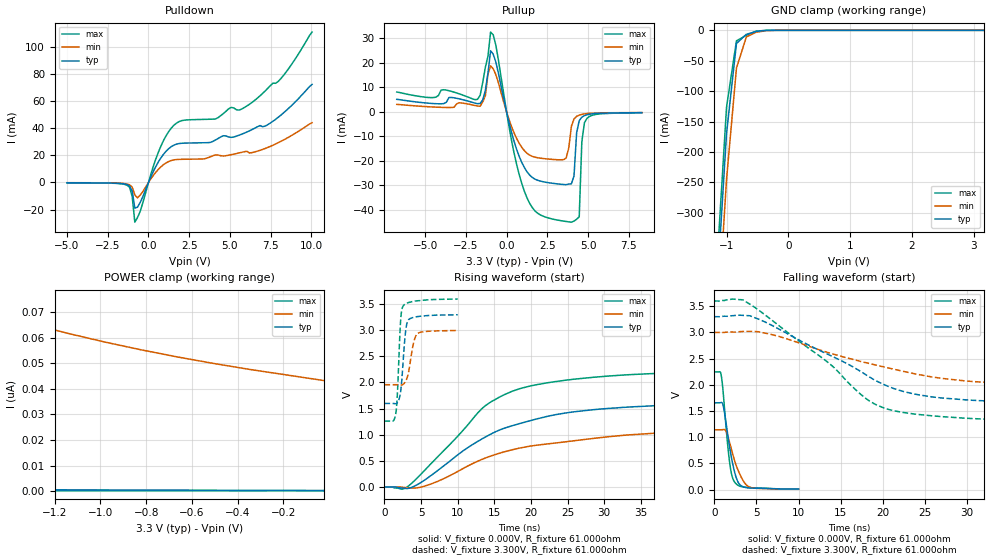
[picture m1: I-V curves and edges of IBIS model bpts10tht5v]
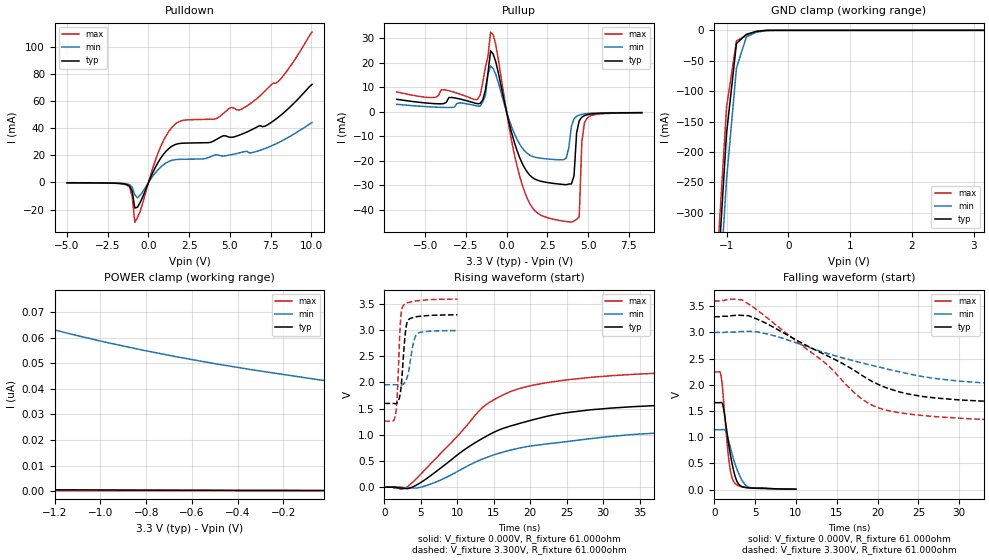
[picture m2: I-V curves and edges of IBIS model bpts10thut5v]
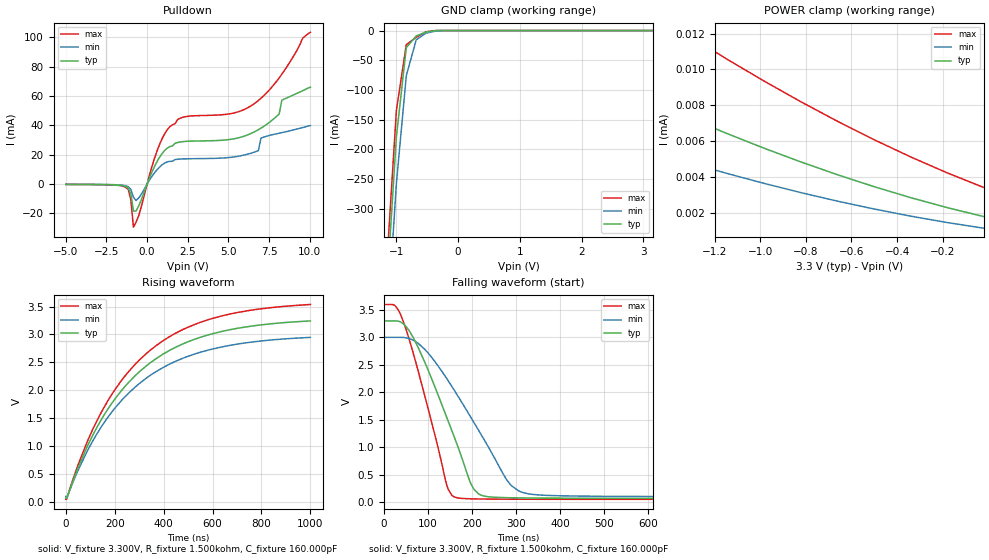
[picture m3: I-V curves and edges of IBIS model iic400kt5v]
[IBIS Ver]  4.0
[File Name]  lpc214x.ibs
[File Rev]  1.0
[Date]   Fri Mar  9 10:51:09 PST 2007
[Source]   Package model from Ansoft Q3D Extractor 7.1.1
[Notes]   IO models Rev 0.20 IBIS Model Design Automation Generation
[Copyright] NXP Semiconductors 2006, 2007. All rights reserved.
|   LPC2141/2142/2144/2146/2148 IBIS Model
[Disclaimer]
| NXP Semiconductors warrants and represents that the IBIS models
| identified herein are owned by NXP Semiconductors (NXP).  The
| models provided are not warranted as fully representing all of the
| operating characteristics and specifications of the semiconductor
| products to which the models relate.  Moreover, unless there is a
| signed, written agreement to the contrary, these models are furnished
| on an "as is" basis without support or warranty of any kind, either
| expressed or implied, regarding the use thereof, and NXP
| specifically disclaims all implied warranties of merchantability and
| fitness of the models for any purpose.
| NXP does not assume any liability arising out of the application
| or use of these IBIS models including infringement of patents and
| copyrights, nor does NXP convey any license under its patents and
| copyrights or the rights of others.
| NXP provides IBIS models as a service to our customers.  You and
| your company shall not distribute, convey, sell, or give these models
| to anyone else without receiving prior written permission from
| NXP.
[Define Package Model]  LQFP64
[Manufacturer]  NXP Semiconductors
[OEM]  NXP Semiconductors
[Description]  LQFP64
|   A full package IBIS Model
|Sim freq : 100 MHz.
|Date : 11/20/06
[Number Of Pins]  64
[Pin Numbers]
pin1   | pin1 = lead1
pin2   | pin2 = lead2
pin3   | pin3 = lead3
pin4   | pin4 = lead4
pin5   | pin5 = lead5
pin6   | pin6 = lead6
pin7   | pin7 = lead7
pin8   | pin8 = lead8
pin9   | pin9 = lead9
pin10   | pin10 = lead10
pin11   | pin11 = lead11
pin12   | pin12 = lead12
pin13   | pin13 = lead13
pin14   | pin14 = lead14
pin15   | pin15 = lead15
pin16   | pin16 = lead16
pin17   | pin17 = lead17
pin18   | pin18 = lead18
pin19   | pin19 = lead19
pin20   | pin20 = lead20
pin21   | pin21 = lead21
pin22   | pin22 = lead22
pin23   | pin23 = lead23
pin24   | pin24 = lead24
pin25   | pin25 = lead25
pin26   | pin26 = lead26
pin27   | pin27 = lead27
pin28   | pin28 = lead28
pin29   | pin29 = lead29
pin30   | pin30 = lead30
pin31   | pin31 = lead31
pin32   | pin32 = lead32
pin33   | pin33 = lead33
pin34   | pin34 = lead34
pin35   | pin35 = lead35
pin36   | pin36 = lead36
pin37   | pin37 = lead37
pin38   | pin38 = lead38
pin39   | pin39 = lead39
pin40   | pin40 = lead40
pin41   | pin41 = lead41
pin42   | pin42 = lead42
pin43   | pin43 = lead43
pin44   | pin44 = lead44
pin45   | pin45 = lead45
pin46   | pin46 = lead46
pin47   | pin47 = lead47
pin48   | pin48 = lead48
pin49   | pin49 = lead49
pin50   | pin50 = lead50
pin51   | pin51 = lead51
pin52   | pin52 = lead52
pin53   | pin53 = lead53
pin54   | pin54 = lead54
pin55   | pin55 = lead55
pin56   | pin56 = lead56
pin57   | pin57 = lead57
pin58   | pin58 = lead58
pin59   | pin59 = lead59
pin60   | pin60 = lead60
pin61   | pin61 = lead61
pin62   | pin62 = lead62
pin63   | pin63 = lead63
pin64   | pin64 = lead64
[Model Data]
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[End Model Data]
[End Package Model]
[Component]   LPC214x
[Manufacturer]  NXP
[Package]
|   typ   min   max
R_pkg   0   0   0  |Values included in pin data
L_pkg   0   0   0  |Values included in pin data
C_pkg   0   0   0  |Values inculded in pin data
[Package Model]  LQFP64
[Pin]   signal_name   model_name   R_pin   L_pin   C_pin
pin1   P0.21   bpts10thut5v   0.1300  4.0559E-9  4.7109E-13
pin2   P0.22   bpts10thut5v   0.1249  3.8553E-9  4.8631E-13
pin3   RTCX1   NC
pin4   P1.19   bpts10thut5v   0.1140  3.4855E-9  4.5269E-13
pin5   RTCX2   NC
pin6   Vss   GND   0.1094  3.2952E-9  4.2167E-13
pin7   V3A   POWER   0.1096  3.2756E-9  4.0402E-13
pin8   P1.18   bpts10thut5v   0.1109  3.2921E-9  3.6808E-13
pin9   P0.25   bpts10thut5v   0.1118  3.3305E-9  3.6694E-013
pin10   D+   usb11f1_iop_hs 0.1126  3.3750E-9  3.9924E-013
pin11   D-   usb11f1_iom_hs 0.1137  3.4080E-9  4.1595E-013
pin12   P1.17   bpts10thut5v   0.1145  3.4513E-9  4.3225E-013
pin13   P0.28   bpts10thut5v   0.1168  3.5314E-9  4.4257E-013
pin14   P0.29   bpts10thut5v   0.1182  3.6136E-9  4.5871E-013
pin15   P0.30   bpts10thut5v   0.1237  3.7941E-9  4.8609E-013
pin16   P1.16   bpts10thut5v   0.1315  4.0543E-9  4.7834E-013
pin17   P0.31OUT   bpts10thut5v   0.1361  4.2525E-9  4.7909E-013
pin18   Vss   GND   0.1370  4.1605E-9  4.9716E-013
pin19   P0.0   bpts10tht5v   0.1359  4.0491E-9  4.5395E-013
pin20   P1.31   bpts10thut5v   0.1359  3.9977E-9  4.7025E-013
pin21   P0.1   bpts10thut5v   0.1368  3.9780E-9  4.6287E-013
pin22   P0.2   iic400kt5v   0.1382  3.9645E-9  4.3275E-013
pin23   V3   POWER   0.1399  3.9938E-9  4.8661E-013
pin24   P1.26   bpts10thut5v   0.1388  3.9783E-9  3.8793E-013
pin25   Vss   GND   0.0849  3.5754E-9  4.5025E-013
pin26   P0.3   iic400kt5v   0.1414  3.9773E-9  4.4598E-013
pin27   P0.4   bpts10thut5v   0.1385  3.9806E-9  4.5362E-013
pin28   P1.25   bpts10thut5v   0.1369  3.9926E-9  4.6653E-013
pin29   P0.5   bpts10thut5v   0.1365  4.0288E-9  4.7531E-013
pin30   P0.6   bpts10thut5v   0.1365  4.0916E-9  4.8687E-013
pin31   P0.7   bpts10thut5v   0.1378  4.1971E-9  4.9554E-013
pin32   P1.24   bpts10thut5v   0.1365  4.2816E-9  4.7853E-013
pin33   P0.8   bpts10thut5v   0.1310  4.0617E-9  4.7309E-013
pin34   P0.9   bpts10thut5v   0.1259  3.8617E-9  4.8581E-013
pin35   P0.10   bpts10thut5v   0.1201  3.6800E-9  4.6639E-013
pin36   P1.23   bpts10thut5v   0.1153  3.5257E-9  4.4746E-013
pin37   P0.11   iic400kt5v   0.1112  3.4101E-9  4.3180E-013
pin38   P0.12   bpts10thut5v   0.1100  3.3561E-9  4.1423E-013
pin39   P0.13   bpts10thut5v   0.1088  3.3002E-9  3.9779E-013
pin40   P1.22   bpts10thut5v   0.1078  3.2747E-9  3.6621E-013
pin41   P0.14   iic400kt5v   0.1076  3.2745E-9  3.6517E-013
pin42   Vss   GND   0.1075  3.2751E-9  3.9548E-013
pin43   V3   POWER   0.1077  3.3057E-9  4.0838E-013
pin44   P1.21   bpts10thut5v   0.1062  3.3049E-9  4.2204E-013
pin45   P0.15   bpts10thut5v   0.1080  3.3717E-9  4.3944E-013
pin46   P0.16   bpts10thut5v   0.1130  3.5156E-9  4.6433E-013
pin47   P0.17   bpts10tht5v   0.1208  3.7554E-9  4.8898E-013
pin48   P1.20   bpts10thut5v   0.1286  4.0340E-9  4.7542E-013
pin49   Vbat   POWER   0.1344  4.2556E-9  4.7786E-013
pin50   Vss   GND   0.1352  4.1540E-9  4.9213E-013
pin51   V3   POWER   0.0836  3.6217E-9  5.4270E-013
pin52   P1.30   bpts10thut5v   0.1370  3.9777E-9  4.7969E-013
pin53   P0.18   bpts10tht5v   0.1349  3.9992E-9  4.5890E-013
pin54   P0.19   bpts10tht5v   0.1360  3.9699E-9  4.5111E-013
pin55   P0.20   bpts10thut5v   0.1381  3.9661E-9  4.4458E-013
pin56   P1.29   bpts10thut5v   0.1408  4.0072E-9  4.2053E-013
pin57   !RESET   bpts10thut5v   0.1433  4.0992E-9  4.1128E-013
pin58   P0.23   bpts10tht5v   0.1380  3.9903E-9  4.3123E-013
pin59   VssA   GND   0.1360  3.9632E-9  4.5084E-013
pin60   P1.28   bpts10thut5v   0.1345  3.9588E-9  4.6165E-013
pin61   XTAL2   NC
pin62   XTAL1   NC
pin63   Vref   POWER   0.1338  4.1409E-9  4.9198E-013
pin64   P1.27   bpts10thut5v   0.1358  4.2774E-9  4.8196E-013
| Models and submodels in the file (5): bpts10tht5v (I/O), bpts10thut5v (I/O), iic400kt5v (I/O_open_drain), usb11f1_iom_hs (I/O), usb11f1_iop_hs (I/O)
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| *   bpts10tht5v  Model   *
[Model]   bpts10tht5v
Model_type   I/O
Polarity   Non-Inverting
Enable   Active-Low
|  Reciever Thresholds
Vinl   = 0.545VV
Vinh   = 1.265VV
| AC Test Load Conditions
Vref   = 0
Cref   = 1.2e-11
Rref   = 1000000000
Vmeas   = 1.4
| [Process Range]   typical   min   max
| C_comp edge width   400.000ps   400.000ps   400.000ps
| C_comp Tstrobe   4.000ps   4.000ps   4.000ps
C_comp   2.882pF   2.754pF   3.016pF
[Temperature Range]   25   125   -40
[Voltage Range]   3.30V   3.00V   3.60V
[GND Clamp Reference]   0.00V   0.00V   0.00V
[Pulldown Reference]   0.00V   0.00V   0.00V
[POWER Clamp Reference]   3.30V   3.00V   3.60V
[Pullup Reference]   3.30V   3.00V   3.60V
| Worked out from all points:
|   slope of the pulldown table from 0 to 0.495 V, typ, clamps not added: 38.6 ohm
|   slope of the pullup table from 0 to 0.495 V, typ, clamps not added: 38.7 ohm
|   GND clamp passes 1 mA (typ) near -0.44 V on its own axis
|   rising waveform, V_fixture 0.000V, R_fixture 61.000ohm: 20-80 % time 13.9ns typ, 18.1ns min, 10.5ns max; typ from 0 V to 1.65 V
|   falling waveform, V_fixture 0.000V, R_fixture 61.000ohm: 20-80 % time 1.06ns typ, 1.41ns min, 788ps max; typ from 1.66 V to 0.008 V
|   rising waveform, V_fixture 3.300V, R_fixture 61.000ohm: 20-80 % time 569ps typ, 787ps min, 437ps max; typ from 1.6 V to 3.29 V
|   falling waveform, V_fixture 3.300V, R_fixture 61.000ohm: 20-80 % time 12.2ns typ, 15ns min, 10.4ns max; typ from 3.3 V to 1.6 V
[GND Clamp]
| ref voltage   0.00V   0.00V   0.00V
|   Voltage   I(typ)   I(min)   I(max)
-5V       -7.936A    -7.958A    -7.931A
-1.16V    -433.2mA   -505.8mA   -392.3mA
-1V       -169.3mA   -244.9mA   -126mA
-840mV    -21.65mA   -62.12mA   -17.29mA
-680mV    -6.579mA   -10.88mA   -8.151mA
-520mV    -1.841mA   -3.127mA   -1.366mA
-360mV    -58.55uA   -596.5uA   -10.53uA
3.16V     300.3pA    45.14nA    134.1pA
[Power Clamp]   | Vtable = Vcc - Vpad
| ref voltage   3.30V   3.00V   3.60V
|   Voltage   I(typ)   I(min)   I(max)
-6.74V    16.52nA    857.8nA    1.18nA
-6.26V    12.33nA    692.5nA    963.8pA
-5.78V    8.96nA     546.5nA    798.2pA
-5.3V     6.516nA    429.9nA    680.5pA
-4.82V    4.749nA    337.5nA    594.2pA
-3.54V    2.1nA      176.9nA    442.2pA
-1.78V    781.7pA    78.68nA    301.1pA
-1.62V    721.7pA    73.79nA    289.6pA
-1.3V     618pA      65.31nA    266.9pA
-820mV    494.3pA    55.22nA    233.5pA
-500mV    427.7pA    49.86nA    211.6pA
-20mV     328.1pA    43.23nA    160.9pA
[Pulldown]
| ref voltage   0.00V   0.00V   0.00V
|   Voltage   I(typ)   I(min)   I(max)
-5V       -226.8uA   -172uA     -259.4uA
-1.32V    -1.578mA   -1.108mA   -2.063mA
-1V       -6.341mA   -3.477mA   -10.45mA
-840mV    -18.89mA   -9.1mA     -29.38mA
-520mV    -15.05mA   -9.482mA   -21.77mA
600mV     15.09mA    9.63mA     22.21mA
1.56V     27.63mA    16.73mA    42.32mA
4.12V     31.49mA    20.45mA    47.01mA
5.08V     33.37mA    20.55mA    55.52mA
6.2V      38.22mA    21.8mA     57.89mA
8.12V     49.75mA    30.36mA    76.76mA
10.04V    72.56mA    44.23mA    111.2mA
[Pullup]   | Vtable = Vcc - Vpad
| ref voltage   3.30V   3.00V   3.60V
|   Voltage   I(typ)   I(min)   I(max)
-6.74V    5.102mA    3.047mA    8.092mA
-1.78V    3.316mA    2.358mA    5.11mA
-1.3V     8.752mA    6.618mA    18.2mA
-980mV    24.92mA    18.76mA    32.55mA
460mV     -12.04mA   -8.591mA   -16.77mA
1.26V     -24.51mA   -16.93mA   -35.2mA
3.5V      -29.67mA   -19.53mA   -44.61mA
3.98V     -29.41mA   -5.895mA   -45.06mA
4.46V     -3.621mA   -1.331mA   -42.82mA
4.62V     -2.179mA   -1.037mA   -12.26mA
4.94V     -1.193mA   -714.9uA   -2.614mA
8.3V      -339.1uA   -299.2uA   -399.9uA
[Ramp]
R_load   = 61.000ohm
|   dV/dt(typ)   dV/dt(min)   dV/dt(max)
dV/dt_r   305.900mV/3.510ns   145.145mV/2.850ns   490.517mV/4.045ns
dV/dt_f   219.141mV/3.115ns   95.446mV/2.510ns   385.597mV/3.650ns
[Rising Waveform]  | cubic spline decimation from 16001 points
V_fixture   = 0.000V
R_fixture   = 61.000ohm
|   Time   V(typ)   V(min)   V(max)
0s        2.719nV    462.7nV    1.218nV
2.365ns   -18.26mV   -1.462mV   -40.39mV
3.085ns   -29.34mV   -13.19mV   2.008mV
6.465ns   232.4mV    64.83mV    463.4mV
13.75ns   954.3mV    553.4mV    1.553V
17.31ns   1.167V     708.3mV    1.824V
20.09ns   1.276V     786.4mV    1.937V
25.98ns   1.44V      886.4mV    2.063V
37.81ns   1.561V     1.037V     2.177V
80ns      1.65V      1.132V     2.242V
[Falling Waveform]  | cubic spline decimation from 2001 points
V_fixture   = 0.000V
R_fixture   = 61.000ohm
|   Time   V(typ)   V(min)   V(max)
0s        1.656V     1.141V     2.245V
815ps     1.661V     1.141V     2.196V
1.14ns    1.544V     1.146V     1.714V
1.44ns    1.234V     1.103V     1.128V
1.775ns   861.6mV    927.3mV    589.7mV
2.07ns    588.3mV    751mV      285.4mV
2.43ns    326.3mV    545.9mV    139.7mV
3.07ns    88.13mV    281.3mV    62.36mV
4.29ns    29.3mV     41.45mV    33.11mV
10ns      7.585mV    7.934mV    6.746mV
[Rising Waveform]  | cubic spline decimation from 2001 points
V_fixture   = 3.300V
V_fixture_min = 3.000V
V_fixture_max = 3.600V
R_fixture   = 61.000ohm
|   Time   V(typ)   V(min)   V(max)
0s        1.598V     1.956V     1.261V
1.545ns   1.593V     1.956V     1.409V
1.73ns    1.608V     1.956V     1.697V
2.195ns   1.813V     1.95V      3.166V
2.505ns   2.318V     1.96V      3.451V
2.91ns    3.005V     2.029V     3.505V
3.29ns    3.199V     2.198V     3.526V
4.025ns   3.244V     2.786V     3.551V
4.51ns    3.258V     2.932V     3.56V
10ns      3.293V     2.992V     3.593V
[Falling Waveform]  | cubic spline decimation from 16001 points
V_fixture   = 3.300V
V_fixture_min = 3.000V
V_fixture_max = 3.600V
R_fixture   = 61.000ohm
|   Time   V(typ)   V(min)   V(max)
0s        3.3V       3V         3.6V
3.445ns   3.325V     3.018V     3.619V
7.415ns   3.086V     2.935V     3.162V
13.46ns   2.584V     2.618V     2.432V
18.01ns   2.189V     2.421V     1.736V
19.39ns   2.06V      2.368V     1.604V
21.92ns   1.896V     2.275V     1.485V
26.97ns   1.748V     2.123V     1.392V
37.59ns   1.661V     2.009V     1.313V
80ns      1.602V     1.959V     1.263V
| bpts10thut5v
|   Bidirectional Pad
|   Plain Input
|   3state Output
|   10 ns Slew Rate Control
|   TTL with Hystersis
|   Pull Up
|   5 V Tolerant
[Model]   bpts10thut5v
Model_type   I/O
Polarity   Non-Inverting
Enable   Active-Low
|  Reciever Thresholds
Vinl   = 0.545VV
Vinh   = 1.265VV
| AC Test Load Conditions
Vref   = 0
Cref   = 1.2e-11
Rref   = 1000000000
Vmeas   = 1.4
| [Process Range]   typical   min   max
| C_comp edge width   400.000ps   400.000ps   400.000ps
| C_comp Tstrobe   4.000ps   4.000ps   4.000ps
C_comp   2.882pF   2.755pF   3.017pF
[Temperature Range]   25   125   -40
[Voltage Range]   3.30V   3.00V   3.60V
[GND Clamp Reference]   0.00V   0.00V   0.00V
[Pulldown Reference]   0.00V   0.00V   0.00V
[POWER Clamp Reference]   3.30V   3.00V   3.60V
[Pullup Reference]   3.30V   3.00V   3.60V
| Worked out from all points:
|   slope of the pulldown table from 0 to 0.495 V, typ, clamps not added: 38.6 ohm
|   slope of the pullup table from 0 to 0.495 V, typ, clamps not added: 38.7 ohm
|   GND clamp passes 1 mA (typ) near -0.44 V on its own axis
|   rising waveform, V_fixture 0.000V, R_fixture 61.000ohm: 20-80 % time 13.9ns typ, 18ns min, 10.4ns max; typ from 0.001 V to 1.65 V
|   falling waveform, V_fixture 0.000V, R_fixture 61.000ohm: 20-80 % time 1.06ns typ, 1.42ns min, 789ps max; typ from 1.66 V to 0.009 V
|   rising waveform, V_fixture 3.300V, R_fixture 61.000ohm: 20-80 % time 568ps typ, 786ps min, 435ps max; typ from 1.6 V to 3.29 V
|   falling waveform, V_fixture 3.300V, R_fixture 61.000ohm: 20-80 % time 12.2ns typ, 15ns min, 10.4ns max; typ from 3.3 V to 1.6 V
[GND Clamp]
| ref voltage   0.00V   0.00V   0.00V
|   Voltage   I(typ)   I(min)   I(max)
-5V       -7.936A    -7.958A    -7.931A
-1.16V    -433.2mA   -505.8mA   -392.3mA
-1V       -169.3mA   -244.9mA   -126mA
-840mV    -21.68mA   -62.13mA   -17.32mA
-680mV    -6.6mA     -10.9mA    -8.182mA
-520mV    -1.87mA    -3.149mA   -1.413mA
-360mV    -102.1uA   -619.8uA   -80.45uA
3.16V     297.4pA    45.14nA    130.5pA
[Power Clamp]   | Vtable = Vcc - Vpad
| ref voltage   3.30V   3.00V   3.60V
|   Voltage   I(typ)   I(min)   I(max)
-6.74V    16.53nA    857.8nA    1.186nA
-6.26V    12.34nA    692.5nA    969.7pA
-5.78V    8.966nA    546.5nA    803.5pA
-5.3V     6.521nA    429.9nA    685.1pA
-4.82V    4.753nA    337.5nA    598.2pA
-3.54V    2.102nA    176.9nA    444.5pA
-1.78V    781.9pA    78.68nA    301.1pA
-1.62V    721.7pA    73.79nA    289.4pA
-1.3V     617.5pA    65.31nA    266.3pA
-820mV    493.2pA    55.22nA    232.2pA
-500mV    426pA      49.86nA    209.8pA
-20mV     325.5pA    43.23nA    158.2pA
[Pulldown]
| ref voltage   0.00V   0.00V   0.00V
|   Voltage   I(typ)   I(min)   I(max)
-5V       -226.8uA   -172uA     -259.4uA
-1.32V    -1.578mA   -1.108mA   -2.063mA
-1V       -6.341mA   -3.477mA   -10.45mA
-840mV    -18.89mA   -9.1mA     -29.38mA
-520mV    -15.05mA   -9.482mA   -21.77mA
600mV     15.09mA    9.63mA     22.21mA
1.56V     27.63mA    16.73mA    42.32mA
4.12V     31.49mA    20.45mA    47.01mA
5.08V     33.37mA    20.55mA    55.52mA
6.2V      38.22mA    21.8mA     57.89mA
8.12V     49.75mA    30.36mA    76.76mA
10.04V    72.56mA    44.23mA    111.2mA
[Pullup]   | Vtable = Vcc - Vpad
| ref voltage   3.30V   3.00V   3.60V
|   Voltage   I(typ)   I(min)   I(max)
-6.74V    5.102mA    3.047mA    8.092mA
-1.78V    3.316mA    2.358mA    5.11mA
-1.3V     8.752mA    6.618mA    18.2mA
-980mV    24.92mA    18.76mA    32.55mA
460mV     -12.04mA   -8.591mA   -16.77mA
1.26V     -24.51mA   -16.93mA   -35.2mA
3.5V      -29.67mA   -19.53mA   -44.61mA
3.98V     -29.41mA   -5.895mA   -45.06mA
4.46V     -3.621mA   -1.331mA   -42.82mA
4.62V     -2.179mA   -1.037mA   -12.26mA
4.94V     -1.193mA   -714.9uA   -2.614mA
8.3V      -339.1uA   -299.2uA   -399.9uA
[Ramp]
R_load   = 61.000ohm
|   dV/dt(typ)   dV/dt(min)   dV/dt(max)
dV/dt_r   306.458mV/3.515ns   145.450mV/2.865ns   491.498mV/4.055ns
dV/dt_f   219.141mV/3.115ns   95.446mV/2.510ns   385.597mV/3.650ns
[Rising Waveform]  | cubic spline decimation from 16001 points
V_fixture   = 0.000V
R_fixture   = 61.000ohm
|   Time   V(typ)   V(min)   V(max)
0s        970.7uV    817.2uV    1.159mV
2.365ns   -17.13mV   -644.9uV   -37.02mV
3.215ns   -25.21mV   -13.15mV   18.29mV
6.515ns   239.9mV    69.07mV    474mV
13.58ns   943.6mV    545.7mV    1.538V
17.24ns   1.167V     707.4mV    1.824V
20.38ns   1.289V     794.1mV    1.949V
28.18ns   1.477V     925.9mV    2.096V
37.37ns   1.56V      1.035V     2.177V
80ns      1.652V     1.133V     2.244V
[Falling Waveform]  | cubic spline decimation from 2001 points
V_fixture   = 0.000V
R_fixture   = 61.000ohm
|   Time   V(typ)   V(min)   V(max)
0s        1.659V     1.142V     2.247V
815ps     1.663V     1.142V     2.198V
1.11ns    1.572V     1.147V     1.776V
1.41ns    1.27V      1.115V     1.188V
1.78ns    859.1mV    926mV      587mV
2.045ns   612mV      767.6mV    306.8mV
2.435ns   325.7mV    545.2mV    142.9mV
2.995ns   103.8mV    311.2mV    71.31mV
4.125ns   34.19mV    54.7mV     39.1mV
10ns      8.903mV    9.047mV    8.293mV
[Rising Waveform]  | cubic spline decimation from 2001 points
V_fixture   = 3.300V
V_fixture_min = 3.000V
V_fixture_max = 3.600V
R_fixture   = 61.000ohm
|   Time   V(typ)   V(min)   V(max)
0s        1.6V       1.956V     1.263V
1.545ns   1.595V     1.956V     1.412V
1.73ns    1.61V      1.956V     1.7V
2.205ns   1.825V     1.95V      3.189V
2.555ns   2.422V     1.964V     3.464V
2.865ns   2.953V     2.017V     3.503V
3.105ns   3.149V     2.096V     3.518V
3.94ns    3.241V     2.736V     3.549V
4.46ns    3.257V     2.925V     3.559V
10ns      3.293V     2.992V     3.593V
[Falling Waveform]  | cubic spline decimation from 16001 points
V_fixture   = 3.300V
V_fixture_min = 3.000V
V_fixture_max = 3.600V
R_fixture   = 61.000ohm
|   Time   V(typ)   V(min)   V(max)
0s        3.3V       3V         3.6V
3.445ns   3.325V     3.018V     3.619V
6.9ns     3.129V     2.956V     3.226V
13.44ns   2.585V     2.619V     2.435V
18.03ns   2.187V     2.42V      1.736V
20.25ns   1.996V     2.336V     1.552V
22.16ns   1.889V     2.266V     1.481V
27.05ns   1.749V     2.121V     1.393V
36.82ns   1.666V     2.012V     1.318V
80ns      1.604V     1.959V     1.265V
| *   iic400kt5v  Model   *
[Model]   iic400kt5v
Model_type   I/O_open_drain
Polarity   Non-Inverting
|  Reciever Thresholds
Vinl   = 0.54V
Vinh   = 1.26V
| AC Test Load Conditions
Vref   = 1.8
Cref   = 1.6e-10
Rref   = 1500
Vmeas   = 0.9
| [Process Range]   typical   min   max
| C_comp edge width   400.000ps   400.000ps   400.000ps
| C_comp Tstrobe   4.000ps   4.000ps   4.000ps
C_comp   2.925pF   2.742pF   3.120pF
[Temperature Range]   25   125   -40
[Voltage Range]   3.30V   3.00V   3.60V
[GND Clamp Reference]   0.00V   0.00V   0.00V
[Pulldown Reference]   0.00V   0.00V   0.00V
[POWER Clamp Reference]   3.30V   3.00V   3.60V
[Pullup Reference]   3.30V   3.00V   3.60V
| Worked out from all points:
|   slope of the pulldown table from 0 to 0.495 V, typ, clamps not added: 38.6 ohm
|   GND clamp passes 1 mA (typ) near -0.42 V on its own axis
|   rising waveform, V_fixture 3.300V, R_fixture 1.500kohm, C_fixture 160.000pF: 20-80 % time 324ns typ, 325ns min, 324ns max; typ from 0.072 V to 3.24 V
|   falling waveform, V_fixture 3.300V, R_fixture 1.500kohm, C_fixture 160.000pF: 20-80 % time 94ns typ, 131ns min, 69.5ns max; typ from 3.3 V to 0.073 V
[GND Clamp]
| ref voltage   0.00V   0.00V   0.00V
|   Voltage   I(typ)   I(min)   I(max)
-5V       -7.947A    -7.97A     -7.942A
-1.16V    -440.7mA   -515.2mA   -399.1mA
-1V       -178.2mA   -256.8mA   -134mA
-840mV    -28.69mA   -76.21mA   -23.89mA
-680mV    -9.178mA   -15.72mA   -11.47mA
-520mV    -2.63mA    -4.336mA   -2.114mA
-360mV    -96.99uA   -842.4uA   -23.45uA
-200mV    -429.5nA   -19.6uA    -17.89nA
3.16V     1.358uA    1.421uA    1.528uA
[Power Clamp]   | Vtable = Vcc - Vpad
| ref voltage   3.30V   3.00V   3.60V
|   Voltage   I(typ)   I(min)   I(max)
-6.74V    55.73uA    41uA       80.36uA
-2.58V    17.33uA    13.66uA    24.05uA
-2.42V    14.99uA    11.65uA    21.88uA
-2.26V    13.23uA    9.883uA    20.29uA
-2.1V     12.06uA    8.446uA    18.76uA
-1.94V    11.02uA    7.433uA    17.28uA
-1.78V    10.02uA    6.694uA    15.84uA
-1.46V    8.132uA    5.373uA    13.09uA
-1.3V     7.244uA    4.761uA    11.78uA
-660mV    4.124uA    2.653uA    7.102uA
-340mV    2.85uA     1.819uA    5.121uA
-20mV     1.796uA    1.148uA    3.418uA
[Pulldown]
| ref voltage   0.00V   0.00V   0.00V
|   Voltage   I(typ)   I(min)   I(max)
-5V       -206.2uA   -158.6uA   -234.8uA
-1.32V    -1.618mA   -1.146mA   -2.111mA
-1V       -6.495mA   -3.626mA   -10.71mA
-840mV    -18.4mA    -8.915mA   -29.31mA
600mV     15.09mA    9.627mA    22.21mA
1.4V      25.54mA    15.5mA     39.06mA
6.52V     35.14mA    21.49mA    54.22mA
6.84V     37.03mA    22.78mA    56.89mA
7V        38.08mA    31.29mA    58.41mA
8.12V     47.74mA    34.63mA    72.33mA
8.28V     57.06mA    35.02mA    74.77mA
10.04V    65.94mA    39.83mA    103.3mA
[Ramp]
R_load   = 60.000ohm
|   dV/dt(typ)   dV/dt(min)   dV/dt(max)
dV/dt_r   788.763mV/900.000ps   473.417mV/1.400ns   1.169V/600.000ps
dV/dt_f   786.905mV/141.550ns   470.796mV/185.500ns   1.168V/106.950ns
[Rising Waveform]  | cubic spline decimation from 20001 points
V_fixture   = 3.300V
V_fixture_min = 3.000V
V_fixture_max = 3.600V
R_fixture   = 1.500kohm
C_fixture   = 160.000pF
|   Time   V(typ)   V(min)   V(max)
0s        72.35mV    102.2mV    53.86mV
7.05ns    103.3mV    108.9mV    104.9mV
85.25ns   972.2mV    891.8mV    1.056V
165.3ns   1.619V     1.476V     1.763V
255.1ns   2.134V     1.943V     2.326V
343.8ns   2.488V     2.264V     2.713V
445.7ns   2.764V     2.514V     3.015V
602.9ns   3.017V     2.743V     3.291V
777.6ns   3.16V      2.873V     3.447V
1us       3.242V     2.948V     3.536V
[Falling Waveform]  | cubic spline decimation from 20001 points
V_fixture   = 3.300V
V_fixture_min = 3.000V
V_fixture_max = 3.600V
R_fixture   = 1.500kohm
C_fixture   = 160.000pF
|   Time   V(typ)   V(min)   V(max)
0s        3.297V     2.998V     3.595V
25.95ns   3.297V     2.998V     3.565V
43.75ns   3.245V     2.996V     3.285V
92.55ns   2.544V     2.779V     1.93V
141.7ns   1.557V     2.257V     332.8mV
160.5ns   1.163V     2.023V     94.14mV
213.7ns   158.7mV    1.322V     60.58mV
281.6ns   83.47mV    374.7mV    56.44mV
316.9ns   79.14mV    173.6mV    55.64mV
1us       72.53mV    102.8mV    53.92mV
